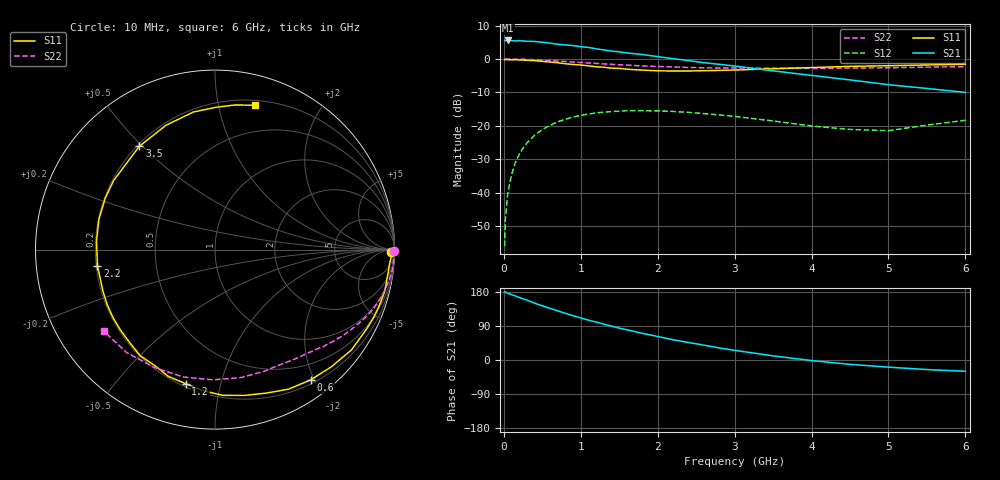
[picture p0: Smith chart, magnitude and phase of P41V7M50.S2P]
! SIEMENS Small Signal Semiconductors
! BFP182
! Si NPN RF Bipolar Junction Transistor in SOT143
! VCE = 1.75 V  IC = 0.5 mA
! Common Emitter S-Parameters:  March  1996
# GHz  S  MA  R  50
!  f  S11  S21  S12  S22
! GHz  MAG  ANG  MAG  ANG  MAG  ANG  MAG  ANG
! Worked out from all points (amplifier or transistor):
!   36 points, 10 MHz to 6 GHz, reference 50 ohm
!   highest |S21| = 5.5 dB at 50 MHz (marker M1)
!   |S21| within 3 dB of that: start of sweep to 1.351 GHz
!   unconditionally stable (mu >= 1): 2.939 GHz to end of sweep
!   at 250 MHz: K = 0.10, MSG = 16.0 dB, |S12| = -26.6 dB
!   at 1.4 GHz: K = 0.51, MSG = 9.0 dB, |S12| = -15.7 dB
!   at 6 GHz: K = 1.25, MAG = 1.2 dB, |S12| = -18.3 dB
!   S11 on the Smith chart (normalised r, x): 10 MHz: 62, -51; 600 MHz: 0.25, -1.95; 1.2 GHz: 0.22, -0.78; 2.2 GHz: 0.21, -0.07; 3.5 GHz: 0.21, +0.49; 6 GHz: 0.24, +1.29
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0.01  0.9809 -0.9  1.879 179.7  0.0016 79.0  0.9999 -0.3
0.02  0.9846 -1.9  1.876 179.3  0.004 87.2  0.9978 -0.6
0.05  0.976 -4.5  1.891 176.3  0.0097 89.3  0.9983 -1.6
0.1  0.9724 -9.0  1.874 172.6  0.0187 83.1  0.9976 -3.4
0.15  0.9737 -13.9  1.861 168.9  0.0285 80.1  0.9952 -5.0
0.2  0.9675 -18.4  1.882 165.0  0.0378 77.9  0.9936 -6.7
0.3  0.9545 -27.2  1.836 158.1  0.0559 72.3  0.9848 -10.0
0.4  0.9438 -36.3  1.828 150.1  0.0726 66.3  0.9744 -13.2
0.6  0.9005 -53.7  1.723 136.2  0.1024 55.2  0.9479 -19.1
0.9  0.8286 -78.7  1.585 116.9  0.1358 40.1  0.9005 -27.1
1.1  0.7885 -95.0  1.488 105.1  0.1507 31.2  0.871 -31.8
1.2  0.7646 -102.3  1.419 100.0  0.1564 26.9  0.8581 -34.1
1.5  0.7234 -125.1  1.281 84.2  0.166 16.3  0.8194 -39.9
1.7  0.6919 -139.5  1.199 75.1  0.1687 10.0  0.7971 -43.6
2.2  0.661 -172.1  1.011 53.5  0.1646 -3.2  0.76 -52.4
2.8  0.6752 154.9  0.833 31.9  0.1462 -14.4  0.7325 -63.6
3.5  0.7136 126.2  0.665 10.9  0.1186 -20.9  0.7274 -78.7
4  0.7447 111.5  0.569 -1.5  0.0998 -18.3  0.7258 -90.9
4.5  0.7761 98.9  0.487 -11.5  0.0887 -11.0  0.7314 -103.9
5  0.793 89.6  0.413 -18.9  0.0849 3.9  0.7384 -117.2
5.5  0.8142 81.9  0.363 -25.2  0.1029 11.3  0.7557 -130.7
6  0.8341 74.5  0.317 -29.8  0.1213 13.1  0.7682 -143.8
